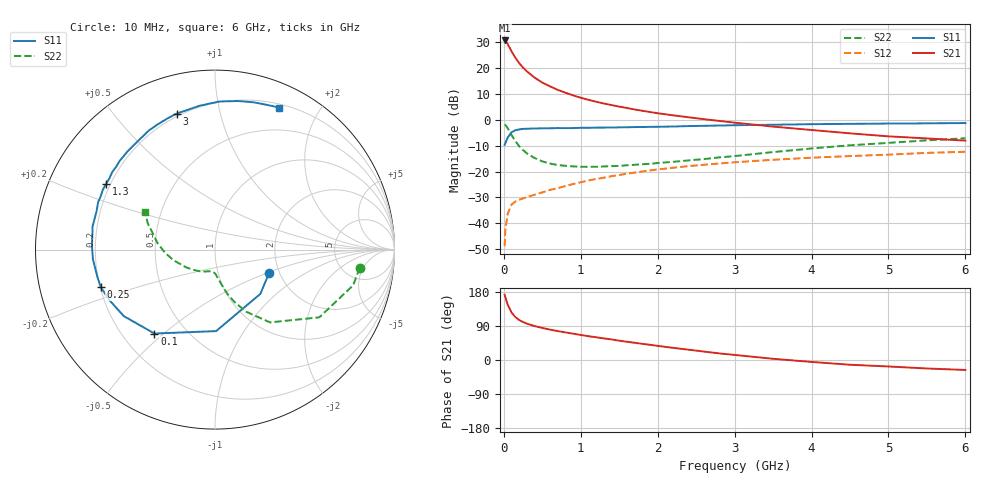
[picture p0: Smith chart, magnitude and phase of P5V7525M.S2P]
! SIEMENS Small Signal Semiconductors
! BFP183
! Si NPN RF Bipolar Junction Transistor in SOT143
! VCE = 0.75 V  IC = 25 mA
! Common Emitter S-Parameters:  March  1996
# GHz  S  MA  R  50
!  f  S11  S21  S12  S22
! GHz  MAG  ANG  MAG  ANG  MAG  ANG  MAG  ANG
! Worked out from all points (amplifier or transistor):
!   36 points, 10 MHz to 6 GHz, reference 50 ohm
!   highest |S21| = 30.7 dB at 10 MHz (marker M1)
!   |S21| within 3 dB of that: start of sweep to 78.48 MHz
!   unconditionally stable (mu >= 1): start of sweep to 12.41 MHz; 336.9 MHz to end of sweep
!   at 250 MHz: K = 0.82, MSG = 25.3 dB, |S12| = -30.4 dB
!   at 1.4 GHz: K = 1.59, MAG = 9.2 dB, |S12| = -21.8 dB
!   at 6 GHz: K = 1.30, MAG = -1.1 dB, |S12| = -12.3 dB
!   S11 on the Smith chart (normalised r, x): 10 MHz: 1.77, -0.51; 100 MHz: 0.33, -0.47; 250 MHz: 0.20, -0.15; 1.3 GHz: 0.18, +0.27; 3 GHz: 0.19, +0.74; 6 GHz: 0.24, +1.53
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0.01  0.3282 -23.2  34.42 172.5  0.0036 79.4  0.8124 -7.2
0.02  0.3532 -44.3  33.72 165.5  0.0075 77.1  0.795 -14.5
0.05  0.4541 -89.2  29.35 145.9  0.0152 62.8  0.6929 -33.0
0.1  0.5766 -125.8  21.17 125.2  0.023 46.8  0.5086 -52.9
0.15  0.6288 -143.9  15.93 113.2  0.0263 41.5  0.3875 -63.3
0.2  0.6536 -154.8  12.51 105.5  0.0285 40.1  0.3096 -69.8
0.25  0.6703 -162.0  10.24 100.1  0.0302 39.6  0.2596 -74.0
0.3  0.6733 -167.8  8.677 96.0  0.032 40.7  0.225 -76.8
0.4  0.6824 -175.5  6.577 89.5  0.0356 43.5  0.1827 -81.1
0.5  0.6858 178.3  5.267 84.6  0.0395 45.7  0.1574 -84.6
0.6  0.6879 173.6  4.456 80.2  0.0441 47.3  0.1428 -87.4
0.7  0.6941 169.2  3.809 76.3  0.0477 49.9  0.134 -89.6
0.9  0.6939 161.8  2.98 69.5  0.0574 51.6  0.126 -94.5
1.1  0.7024 155.3  2.443 62.8  0.0672 52.4  0.1232 -100.3
1.3  0.709 148.9  2.072 56.9  0.076 52.0  0.1256 -105.3
1.7  0.7258 136.9  1.589 45.4  0.0957 50.0  0.1351 -115.4
2.2  0.7438 124.3  1.225 32.1  0.1186 45.9  0.1544 -130.5
3  0.7874 105.7  0.884 13.4  0.1511 37.8  0.1994 -153.4
3.5  0.8055 96.3  0.741 3.2  0.1691 32.8  0.2383 -165.5
4.5  0.8379 81.1  0.549 -12.5  0.1993 22.7  0.3225 173.5
5.5  0.8566 70.3  0.438 -22.4  0.2297 13.7  0.4017 158.8
6  0.8686 65.6  0.397 -26.3  0.2416 8.6  0.4407 152.0
